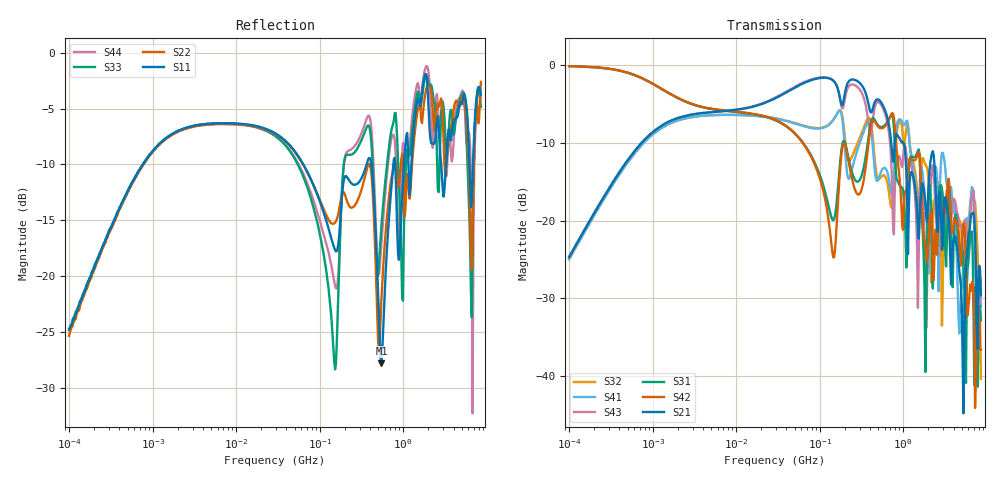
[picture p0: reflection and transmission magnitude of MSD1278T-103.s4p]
# MHz S MA R 50
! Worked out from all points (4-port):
!   498 points, 100 kHz to 8.5 GHz, reference 50 ohm
!   strongest paths, dB at 100 kHz, 1.698 MHz, 29.49 MHz, 500.7 MHz, 8.5 GHz:
!     S21: -24.7, -7.1, -4.2, -4.4, -29.6
!     S42: -0.1, -3.8, -7.0, -7.9, -36.6
!     S31: -0.1, -3.8, -7.1, -7.7, -32.8
!     S43: -24.6, -7.1, -4.1, -4.7, -27.6
!     S41: -24.9, -7.4, -6.8, -14.7, -31.0
!     S32: -24.9, -7.4, -6.8, -14.6, -40.3
!   lowest |S11| = -27.8 dB at 548.6 MHz (marker M1), VSWR 1.08, Z = 52 - j3.61 ohm
!   |S11| at or under -10 dB: 414.5 MHz to 762 MHz (347.5 MHz wide, 59.1 % of centre); 2.843 GHz to 3.261 GHz (417.9 MHz wide, 13.7 % of centre); 6.202 GHz to 6.841 GHz (639.7 MHz wide, 9.81 % of centre)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
0.1  0.058 80.8  0.05832 81.4  0.9879 -3.4  0.05683 -98.9
     0.05832 81.4  0.05395 81.9  0.05662 -98.8  0.9884 -3.4
     0.9879 -3.4  0.05662 -98.8  0.0573 82.3  0.05855 81.3
     0.05683 -98.9  0.9884 -3.4  0.05855 81.3  0.05716 83.4
90.29583  0.2396 -65.3  0.8201 -8.9  0.2263 -78.3  0.3916 86.9
          0.8201 -8.9  0.2406 -69.4  0.395 83.9  0.2195 -79.2
          0.2263 -78.3  0.395 83.9  0.1833 -63.6  0.8276 -12.3
          0.3916 86.9  0.2195 -79.2  0.8276 -12.3  0.2011 -57.1
548.5512  0.04062 -58.6  0.5738 -100.5  0.4011 -17.4  0.2089 -43.8
          0.5738 -100.5  0.07877 -10.9  0.1928 -56.5  0.3928 -18.2
          0.4011 -17.4  0.1928 -56.5  0.168 -24.3  0.5532 -111.6
          0.2089 -43.8  0.3928 -18.2  0.5532 -111.6  0.1413 -29.1
1926.311  0.7561 -179.9  0.09932 170.2  0.07864 -132.9  0.0938 94.2
          0.09932 170.2  0.7086 -154.8  0.2195 116.4  0.05459 143.0
          0.07864 -132.9  0.2195 116.4  0.7793 163.5  0.03595 -144.8
          0.0938 94.2  0.05459 143.0  0.03595 -144.8  0.8706 -177.3
2776.003  0.3492 93.3  0.1508 27.4  0.1685 84.7  0.1923 135.9
          0.1508 27.4  0.6058 106.1  0.107 44.9  0.1096 82.2
          0.1685 84.7  0.107 44.9  0.4092 91.3  0.1606 13.8
          0.1923 135.9  0.1096 82.2  0.1606 13.8  0.4877 96.9
6920.76  0.3573 25.0  0.1125 1.6  0.03198 -57.8  0.1325 -10.4
         0.1125 1.6  0.2631 20.6  0.1378 17.6  0.03622 -21.7
         0.03198 -57.8  0.1378 17.6  0.2579 45.2  0.1569 27.2
         0.1325 -10.4  0.03622 -21.7  0.1569 27.2  0.1597 5.8
8500  0.6483 -56.6  0.03313 -113.3  0.0229 -113.1  0.0283 -179.3
      0.03313 -113.3  0.741 -41.9  0.009622 98.9  0.01477 -135.8
      0.0229 -113.1  0.009622 98.9  0.5718 -51.8  0.04181 -68.9
      0.0283 -179.3  0.01477 -135.8  0.04181 -68.9  0.6243 -55.2
